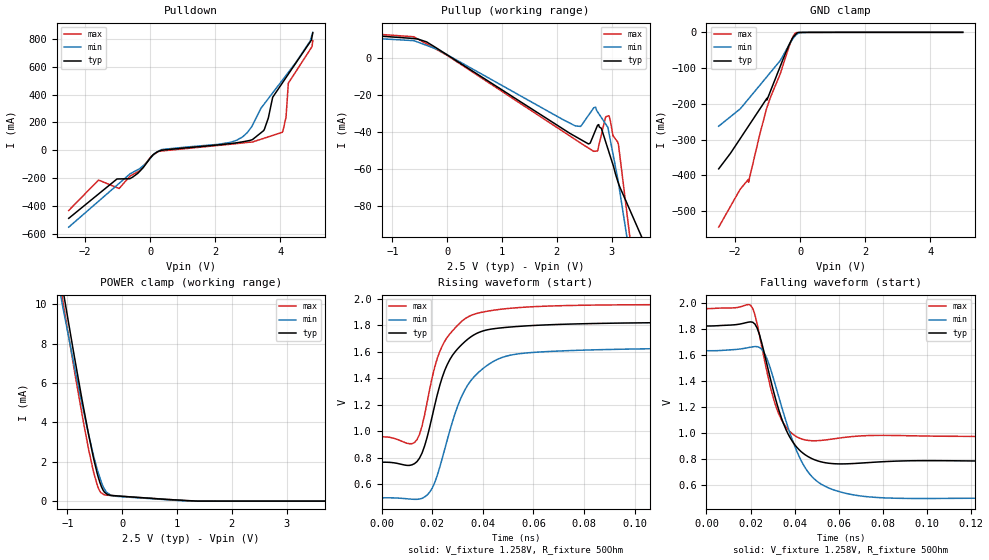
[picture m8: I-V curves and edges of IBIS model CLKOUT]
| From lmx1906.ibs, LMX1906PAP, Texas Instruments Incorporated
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|   Model CLKOUT
[Model]   CLKOUT
Model_type   Output
Polarity   Non-Inverting
Vmeas = 1.25
Vref = 1.25
Cref = 2pF
Rref = 50
|   typ   min   max
C_comp   0.28pF   0.27pF   0.288pF
[Voltage Range]   2.5   2.4   2.6
[Temperature Range]   27   105   -40
[Pullup Reference]   2.5   2.4   2.6
[Pulldown Reference]   0   0   0
[Power Clamp Reference]   2.5   2.4   2.6
[GND Clamp Reference]   0   0   0
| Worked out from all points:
|   slope of the pulldown table from 0 to 0.375 V, typ, clamps not added: 6.51 ohm
|   slope of the pullup table from 0 to 0.375 V, typ, clamps not added: 52.7 ohm
|   GND clamp passes 1 mA (typ) near -0.08 V on its own axis
|   POWER clamp passes 1 mA (typ) near -0.41 V on its own axis
|   falling waveform, V_fixture 1.258V, R_fixture 50Ohm: 20-80 % time 11.3ps typ, 14.7ps min, 8.55ps max; typ from 1.82 V to 0.766 V
|   rising waveform, V_fixture 1.258V, R_fixture 50Ohm: 20-80 % time 11.3ps typ, 13.4ps min, 10.6ps max; typ from 0.766 V to 1.82 V
[Pulldown]
|   Voltage   I(typ)   I(min)   I(max)
-2.5V     -488.4mA   -551.8mA   -432.1mA
-1.584V   -313.9mA   -365.9mA   -213.7mA
-951.9mV  -205.7mA   -237.7mA   -274.5mA
250.8mV   -8.257mA   -7.638mA   -9.567mA
2.469V    48.07mA    57.22mA    43.17mA
3.146V    76.45mA    179.5mA    59.38mA
3.503V    146.2mA    330.7mA    86.37mA
3.768V    380.5mA    411.7mA    106.4mA
4.062V    481.8mA    501.7mA    128.7mA
4.177V    521.8mA    537.1mA    236.6mA
4.249V    546.4mA    558.9mA    481.6mA
5V        842.5mA    846.4mA    786.4mA
[GND Clamp]
|   Voltage   I(typ)   I(min)   I(max)
-2.5V     -381.8mA   -262.5mA   -544.8mA
-1.854V   -299.2mA   -215mA     -441mA
-1.587V   -262.6mA   -186.5mA   -411.3mA
-1.584V   -262.2mA   -186.2mA   -411.5mA
-1.584V   -262.2mA   -186.2mA   -419.3mA
-1.234V   -214.1mA   -147.7mA   -284.1mA
-1.019V   -184.6mA   -124.2mA   -210.7mA
-609.4mV  -95.39mA   -79.18mA   -116.3mA
-351.6mV  -38.08mA   -36.94mA   -43.83mA
-147.6mV  -6.892mA   -9.592mA   -2.495mA
184.2mV   -210.7uA   -193.8uA   -208.8uA
5V        0A         0A         0A
[Pullup]
|   Voltage   I(typ)   I(min)   I(max)
-2.5V     14.41mA    12.37mA    15.26mA
-611.2mV  10.36mA    9.226mA    11.33mA
2.324V    -42.36mA   -36.7mA    -44mA
2.579V    -46.67mA   -31.09mA   -48.9mA
2.708V    -39.11mA   -26.71mA   -50.56mA
2.812V    -38.16mA   -32.35mA   -41.77mA
2.893V    -45.66mA   -35.95mA   -31.95mA
2.951V    -51.05mA   -40.68mA   -31.41mA
3.027V    -58.08mA   -52.34mA   -42.39mA
3.146V    -69.69mA   -71.68mA   -52.02mA
3.544V    -96.66mA   -147.8mA   -147.8mA
5V        -763.1mA   -740.2mA   -828mA
[POWER Clamp]
|   Voltage   I(typ)   I(min)   I(max)
-2.5V     35.32mA    31.57mA    35.42mA
-1.213V   12.92mA    11.75mA    12.36mA
-1.089V   10.84mA    9.915mA    10.23mA
-1.036V   9.961mA    9.149mA    9.317mA
-852.5mV  6.993mA    6.542mA    6.273mA
-611.2mV  3.344mA    3.338mA    2.582mA
-521.8mV  2.15mA     2.282mA    1.445mA
-449.1mV  1.324mA    1.541mA    747.2uA
-333.2mV  488.6uA    653.4uA    321.9uA
-172mV    284.8uA    267.2uA    277.3uA
1.142V    36.42uA    10.63uA    29.06uA
5V        0A         0A         0A
[Ramp]
R_load = 50
|   typ   min   max
dV/dt_r   0.633158/1.12776e-11   0.680068/1.33682e-11   0.598474/1.06046e-11
dV/dt_f   0.633158/1.12536e-11   0.68503/1.47033e-11   0.598474/8.55005e-12
[Falling Waveform]
V_fixture = 1.258V
V_fixture_min = 1.065V
V_fixture_max = 1.393V
R_fixture = 50Ohm
C_fixture = 0F
|   Time   V(typ)   V(min)   V(max)
0s        1.821V     1.631V     1.955V
19ps      1.851V     1.655V     1.986V
22ps      1.836V     1.663V     1.908V
26ps      1.63V      1.622V     1.588V
31ps      1.285V     1.385V     1.232V
40ps      911.2mV    901.6mV    980mV
46ps      818.8mV    702.3mV    942.1mV
52ps      777.2mV    606.7mV    941.6mV
77ps      774.9mV    503.5mV    980.2mV
1ns       766mV      489.3mV    957.2mV
[Rising Waveform]
V_fixture = 1.258V
V_fixture_min = 1.065V
V_fixture_max = 1.393V
R_fixture = 50Ohm
C_fixture = 0F
|   Time   V(typ)   V(min)   V(max)
0s        766mV      497.3mV    957.2mV
13ps      754.8mV    485.9mV    914.3mV
16ps      834.8mV    493.5mV    1.038V
19ps      1.029V     539.5mV    1.314V
22ps      1.273V     665.8mV    1.547V
25ps      1.46V      866.6mV    1.679V
32ps      1.659V     1.277V     1.833V
45ps      1.774V     1.534V     1.914V
63ps      1.799V     1.597V     1.941V
1ns       1.821V     1.631V     1.955V
